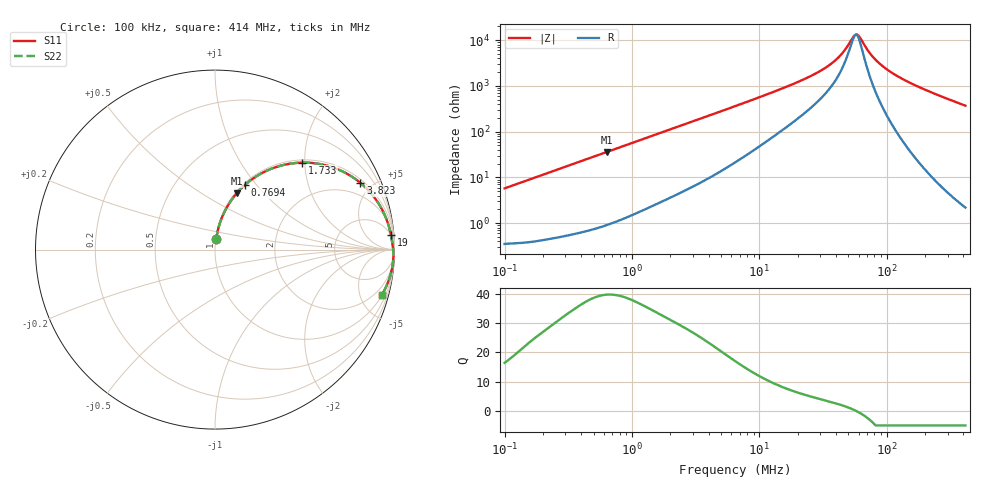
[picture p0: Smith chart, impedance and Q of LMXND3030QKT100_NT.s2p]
! LMXND3030QKT100_NT  S-PARAMETER MODEL  ( Standard Model )
! Model Generated by TAIYO YUDEN Corporation (https://www.yuden.co.jp/en/)
! Version 1.0
! TAIYO YUDEN Control No. 20250724
! Copyright(c) 2025 TAIYO YUDEN CO.,LTD. All Rights Reserved.
! Product Description (link to TY-COMPAS)
! https://ds.yuden.co.jp/TYCOMPAS/or/detail?pn=LMXND3030QKT100MNT&u=M
! Products Name : Inductors
! Characteristics :
!  Inductance : 10 [uH] , SRF(min) : 28 [MHz] , DC Resistance(max) : 0.264 [Ohm]
!  Rated Current : Saturation  700 [m A] , Temp Rise  1080 [m A] (40 [degC])
!  Case Size : 3.0 x 3.0 / 0.118 x 0.118 [mm/inch] , Thickness : 1.5 / 0.059 [mm/inch]
!  (Conditions: Temperature = 25 [degC] , DC Bias Current = 0 [A])
! External Node Assignments :
!  1  o---GGG---o  2
! GND o---------o GND
! Frequency Range : 0.1MHz  -  413.982163MHz  [ 402 STEP ]
# MHz S RI R 50
! Freq[MHz].  S11 Real  S11 Imag  S21 Real  S21 Imag  S12 Real  S12 Imag  S22 Real  S22 Imag
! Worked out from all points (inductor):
!   401 points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, 100 kHz to 414 MHz, reference 50 ohm
!   read as one part in series: L = 9.13 uH near 104.3 kHz
!   highest Q = 39.6 at 637.9 kHz (marker M1), where L = 9.02 uH
!   self-resonance near 56.09 MHz
!   S11 on the Smith chart (normalised r, x): 100 kHz: 1.01, +0.12; 769.4 kHz: 1.02, +0.87; 1.733 MHz: 1.06, +1.95; 3.823 MHz: 1.18, +4.26; 19 MHz: 4, +23; 414 MHz: 1.04, -7.41
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0.1  0.00676 0.0569  0.9932 -0.0569  0.9932 -0.0569  0.00676 0.0569
0.403501  0.0554 0.2154  0.9446 -0.2154  0.9446 -0.2154  0.0554 0.2154
0.637938  0.1218 0.3147  0.8782 -0.3147  0.8782 -0.3147  0.1218 0.3147
0.769415  0.1658 0.3594  0.8342 -0.3594  0.8342 -0.3594  0.1658 0.3594
1.628129  0.457 0.4833  0.543 -0.4833  0.543 -0.4833  0.457 0.4833
1.73307  0.4869 0.4847  0.5131 -0.4847  0.5131 -0.4847  0.4869 0.4847
2.469096  0.6513 0.4596  0.3487 -0.4596  0.3487 -0.4596  0.6513 0.4596
3.823222  0.81 0.3718  0.19 -0.3718  0.19 -0.3718  0.81 0.3718
6.434145  0.9159 0.2497  0.0841 -0.2497  0.0841 -0.2497  0.9159 0.2497
18.99759  0.9798 0.0835  0.0202 -0.0835  0.0202 -0.0835  0.9798 0.0835
25.96183  0.9849 0.0558  0.0151 -0.0558  0.0151 -0.0558  0.9849 0.0558
33.33072  0.9879 0.0369  0.0121 -0.0369  0.0121 -0.0369  0.9879 0.0369
40.20007  0.9897 0.0239  0.0103 -0.0239  0.0103 -0.0239  0.9897 0.0239
46.5076  0.991 0.014  0.00899 -0.014  0.00899 -0.014  0.991 0.014
54.93683  0.9923 0.00277  0.00771 -0.00277  0.00771 -0.00277  0.9923 0.00277
57.27281  0.9926 -9.39e-05  0.00743 9.39e-05  0.00743 9.39e-05  0.9926 -9.39e-05
60.96434  0.993 -0.00443  0.00705 0.00443  0.00705 0.00443  0.993 -0.00443
72.01376  0.9937 -0.0164  0.00625 0.0164  0.00625 0.0164  0.9937 -0.0164
79.9149  0.994 -0.0243  0.00596 0.0243  0.00596 0.0243  0.994 -0.0243
104.7562  0.9938 -0.0467  0.0062 0.0467  0.0062 0.0467  0.9938 -0.0467
180.0045  0.9866 -0.1047  0.0134 0.1047  0.0134 0.1047  0.9866 -0.1047
413.9822  0.9308 -0.2508  0.0692 0.2508  0.0692 0.2508  0.9308 -0.2508
